FUNCTION "SCHALING" : VOID
TITLE =Schaling
AUTHOR : MJO
FAMILY : GEMAAL
NAME : SCHALING
VERSION : 0.1


VAR_INPUT
  In : REAL ;	//Ingangswaarde
  X1 : REAL ;	//X-warde punt 1
  Y1 : REAL ;	//Y-waarde punt 1
  X2 : REAL ;	//X-warde punt 2
  Y2 : REAL ;	//Y-waarde punt 2
  Percent0 : REAL ;	//0% waarde
  Percent100 : REAL ;	//100% waarde
END_VAR
VAR_OUTPUT
  Uit : REAL ;	//Uitgangswaarde
  Percentage : REAL ;	//Uitgangswaarde in %
END_VAR
VAR_TEMP
  A : REAL ;	//Schalingsconstante A
  B : REAL ;	//Schalingsconstante B
  TmpReal : REAL ;
END_VAR
BEGIN
NETWORK
TITLE =Bereken constante A
//Berekenen constante A: A = (Uit2 - Uit1) / (In2 - In1)
//
      L     #X2;
      L     #X1;
      -R    ; //Berekend (In2 - In1)
      T     #TmpReal; //Tijdelijke opslag resultaat
      L     #Y2;
      L     #Y1;
      -R    ; //Berekend (Uit2 - Uit1)
      L     #TmpReal; //Ophalen (Uit2 - Uit1)
      /R    ; //Berekend (In2 - In1)/(Uit2 - Uit1)
      T     #A;
NETWORK
TITLE =Bereken constante B
//Berekenen constante B: B = Uit1 - (A * In1)
//
      L     #A;
      L     #X1;
      *R    ; //Berekend (A * In1)
      T     #TmpReal; //Tijdelijke opslag resultaat
      L     #Y1;
      L     #TmpReal;
      -R    ; //Berekend Uit1 - (A * In1)
      T     #B;
NETWORK
TITLE =Bepaal uitgangswaarde
//
//
      L     #In;
      L     #A;
      *R    ;
      L     #B;
      +R    ;
      T     #Uit;
NETWORK
TITLE =Bepaal percentage
//Voor bepaling van percentage geldt: Y1 ~ 0% en Y2 ~ 100%.
//Uitganspercentage wordt berekend volgens:
//       x % = (#Uit - Y1) * 100 / (Y2 - Y1)
      L     #Percent100;
      L     #Percent0;
      -R    ;
      T     #TmpReal;
      L     #Uit;
      L     #Percent0;
      -R    ;
      L     1.000000e+002;
      *R    ;
      L     #TmpReal;
      /R    ;
      T     #Percentage;
END_FUNCTION

